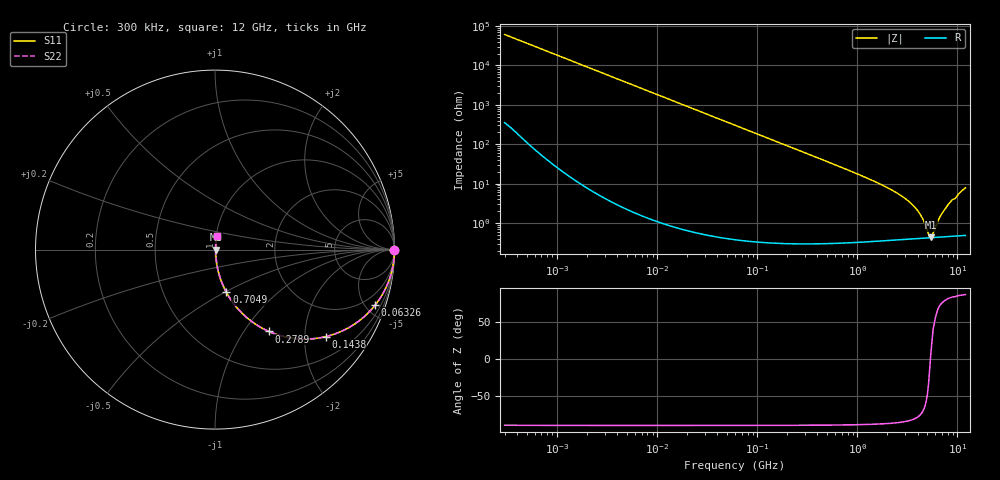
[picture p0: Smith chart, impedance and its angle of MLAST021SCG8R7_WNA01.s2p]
! MLAST021SCG8R7_WNA01  S-PARAMETER MODEL  ( General Type )
! Model Generated by TAIYO YUDEN Corporation (http://www.ty-top.com)
! Version 1.0
! TAIYO YUDEN Control No. 220901
! Copyright(c) 2022 TAIYO YUDEN CO.,LTD. All Rights Reserved.
! Product Description (link to TY-COMPAS)
! https://ds.yuden.co.jp/TYCOMPAS/or/detail?pn=MLAST021SCG8R7CWNA01&u=M
! Products Name : Multilayer Ceramic Capacitors
! Characteristics :
!  Capacitance : 8.7 pF , Rated Voltage : 25V , TCC : CG / C0G
!  Case Size : 0.25 x 0.125 / 0.0098 x 0.0049 [mm/inch] , Thickness : 0.125 / 0.0049 [mm/inch]
!  (Conditions: Temperature = 25 degC , DC Bias Current/Voltage = 0A / 0V)
! External Node Assignments :
!  1  o---| |---o  2
! GND o---------o GND
! Frequency Range : 0.3MHz  -  12000MHz  [ 401 STEP ]
# MHz S RI R 50
! Freq[MHz].  S11 Real  S11 Imag  S21 Real  S21 Imag  S12 Real  S12 Imag  S22 Real  S22 Imag
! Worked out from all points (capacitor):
!   401 points, 300 kHz to 12 GHz, reference 50 ohm
!   read as one part in series: C = 8.7 pF near 316.3 kHz
!   lowest |Z| = 431 mohm at 5.42 GHz (marker M1)
!   series resonance near 5.378 GHz, so ESL is about 100 pH
!   S11 on the Smith chart (normalised r, x): 300 kHz: open; 63.26 MHz: 1.01, -5.78; 143.8 MHz: 1.01, -2.54; 278.9 MHz: 1.01, -1.31; 704.9 MHz: 1.01, -0.51; 12 GHz: 1.01, +0.16
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0.3  1 -0.00164  1.22e-05 0.00164  1.22e-05 0.00164  1 -0.00164
1.769972  0.9999 -0.00967  0.000102 0.00967  0.000102 0.00967  0.9999 -0.00967
10.44266  0.9967 -0.0569  0.00328 0.0569  0.00328 0.0569  0.9967 -0.0569
26.39317  0.9795 -0.1413  0.0205 0.1413  0.0205 0.1413  0.9795 -0.1413
60  0.9026 -0.2959  0.0974 0.2959  0.0974 0.2959  0.9026 -0.2959
63.26471  0.8928 -0.3087  0.1072 0.3087  0.1072 0.3087  0.8928 -0.3087
94.13233  0.7901 -0.4063  0.2099 0.4063  0.2099 0.4063  0.7901 -0.4063
143.8206  0.6174 -0.4848  0.3826 0.4848  0.3826 0.4848  0.6174 -0.4848
278.9009  0.3005 -0.4562  0.6995 0.4562  0.6995 0.4562  0.3005 -0.4562
353.9943  0.2107 -0.4049  0.7893 0.4049  0.7893 0.4049  0.2107 -0.4049
704.9044  0.0636 -0.2381  0.9364 0.2381  0.9364 0.2381  0.0636 -0.2381
2088.533  0.00904 -0.0734  0.991 0.0734  0.991 0.0734  0.00904 -0.0734
2947.191  0.00569 -0.0429  0.9943 0.0429  0.9943 0.0429  0.00569 -0.0429
3740.715  0.00462 -0.0249  0.9954 0.0249  0.9954 0.0249  0.00462 -0.0249
4385.161  0.0043 -0.0137  0.9957 0.0137  0.9957 0.0137  0.0043 -0.0137
5140.631  0.00423 -0.00289  0.9958 0.00289  0.9958 0.00289  0.00423 -0.00289
5420.343  0.00426 0.00047  0.9957 -0.00047  0.9957 -0.00047  0.00426 0.00047
5715.274  0.00431 0.0036  0.9957 -0.0036  0.9957 -0.0036  0.00431 0.0036
6699.894  0.0046 0.0137  0.9954 -0.0137  0.9954 -0.0137  0.0046 0.0137
7648.807  0.00506 0.0234  0.9949 -0.0234  0.9949 -0.0234  0.00506 0.0234
8503.825  0.00571 0.0334  0.9943 -0.0334  0.9943 -0.0334  0.00571 0.0334
12000  0.0108 0.0768  0.9892 -0.0768  0.9892 -0.0768  0.0108 0.0768
